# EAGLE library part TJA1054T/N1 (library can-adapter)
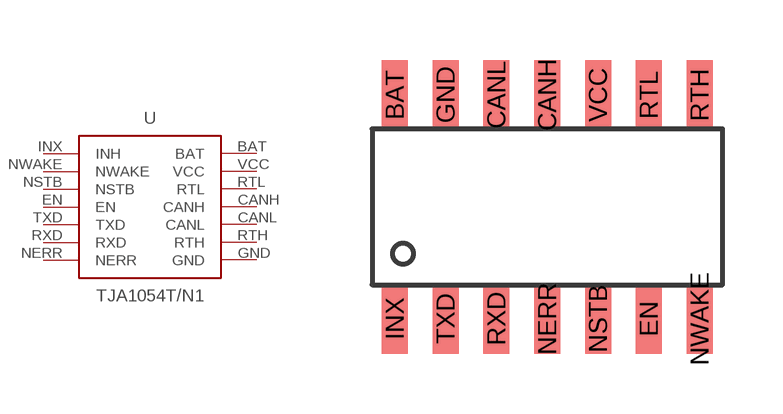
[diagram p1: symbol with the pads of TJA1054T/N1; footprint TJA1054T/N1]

Designator prefix -

## TJA1054T/N1  [TJA1054T/N1]
BAT  BAT  pwr
CANH  CANH
CANL  CANL
EN  EN  in
GND  GND  pwr
INX  INH  out
NERR  NERR  out
NSTB  NSTB  in
NWAKE  NWAKE  in
RTH  RTH
RTL  RTL
RXD  RXD  out
TXD  TXD  in
VCC  VCC  pwr

## Footprint TJA1054T/N1 (pad centres in mm)
smd 0.65 x 1.75: BAT -3.81,2.8; CANH 0,2.8; CANL -1.27,2.8; EN 2.54,-2.8; GND -2.54,2.8; INX -3.81,-2.8; NERR 0,-2.8; NSTB 1.27,-2.8; NWAKE 3.81,-2.8; RTH 3.81,2.8; RTL 2.54,2.8; RXD -1.27,-2.8; TXD -2.54,-2.8; VCC 1.27,2.8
